(* Logix 5000 AddOnInstructionDefinition export MAJ_Yaskawa; software revision 17.00 *)

TYPE Yaskawa_EIP_Servo :   // Yaskawa SigmaLogic Axis Structure v2.4.0
STRUCT
   O : Yaskawa_OUT_to_Servo;
   I : Yaskawa_IN_from_Servo;
   AOI_SB : Yaskawa_AOI_Status_Bits;
END_STRUCT
END_TYPE

TYPE Yaskawa_OUT_to_Servo :   // Structure of data sent out to the Yaskawa SigmaLogic controller v2.4.0
STRUCT
   b00_ServoOn : BOOL;   // Servo On
   b01_Stop : BOOL;   // Stops All Current Motion in Progress
   b02_Home : BOOL;   // Start Homing Process
   b03_MoveStart1 : BOOL;   // Start Current Motion
   b06_SuperImpose : BOOL;
   b07_ServoAlarmReset : BOOL;   // Servo Alarm Reset
   b08_ControllerAlarmReset : BOOL;   // SigmaLogic Alarm Reset
   b09_MoveStart2 : BOOL;   // Start Second Motion (Blended Move)
   b10_MoveAbort : BOOL;   // Abort Current Move
   b11_MovePause : BOOL;   // Pause Current Move
   b12_SeqPause : BOOL;   // Indexing Sequence Pause
   b13_SeqResume : BOOL;   // Indexing Sequence Resume
   b14_SeqCancel : BOOL;   // Indexing Sequence Cancel
   b15_AbsEncoderReset : BOOL;   // Absolute Encoder Reset
   b16_SeqStart : BOOL;   // Start Indexing Sequence
   b17_SeqEditSpeed : BOOL;   // Enter Edit Speed
   b18_SeqEditDistance : BOOL;   // Enter Distance Edit
   b19_PLSEnable : BOOL;   // Enable PLS execution
   b20_PLSActivateOutput1 : BOOL;   // Activate PLS output1 switch logic
   b21_PLSActivateOutput2 : BOOL;   // Activate PLS output2 switch logic
   b22_PLSActivateOutput3 : BOOL;   // Activate PLS output3 switch logic
   b23_PLSActivateOutput4 : BOOL;   // Activate PLS output4 switch logic
   b24_SetClock : BOOL;   // Set the remote controller clock with data provided by the PLC
   RebootController : BOOL;
   UseExternalEncoder : BOOL;   // Use External Encoder when executing MAHSP_Yaskawa
   b32_HeatbeatAnswer : BOOL;   // Heartbeat Answer
   BrakeBypassRequest : BOOL;
   SetFwdTorqueLimit : BOOL;
   SetRevTorqueLimit : BOOL;
   TorqueLimit : DINT;
   TorqueRamp : DINT;
   HomeMethod : INT;
   HomeSpeed : DINT;
   HomeAccDec : DINT;   // Home Move Acceleration/Deceleration Rate
   HomeBackOffDistance : DINT;
   HomeCreepSpeed : DINT;
   HomeCreepDistanceLimit : DINT;
   HomeCreepTimeLimit : DINT;
   HomeOffsetDistance : DINT;
   HomeOffsetSpeed : DINT;
   HomePostion : DINT;
   HomeTorque : DINT;
   HomeInputNo : DINT;
   HomeApproachTimeLimit : DINT;
   HomeApproachDistLimit : DINT;
   HomeDirection : INT;
   HomeSwitchMode : INT;
   MoveType : INT;
   MoveDirection : INT;
   MoveAccel1 : DINT;
   MoveAccel2 : DINT;
   MoveDecel1 : DINT;
   MoveDecel2 : DINT;
   MoveSpeed1 : DINT;
   MoveSpeed2 : DINT;
   MoveDistance1 : DINT;
   MoveDistance2 : DINT;
   MovePosition1 : DINT;
   MovePosition2 : DINT;
   RegistrationDistance : DINT;
   GearNumerator : DINT;
   GearDenominator : DINT;
   SuperImposeDistance : DINT;
   Resolution : INT;
   RegistrationDirection : INT;
   TuningLevel : INT;
   SequenceStep : INT;   // Staring Sequence Step Number
   SequenceEditStep : INT;   // Sequence Step Number to Edit
   FlagCommandBits1 : DINT;   // Flag Commands. 1..64 are General Flags, Bits 0..31 correspond to Flag 1..32
   FlagCommandBits2 : DINT;   // Flag Commands cont. 1..64 are General Flags, Bits 0..31 correspond to Flag 33..64
   DigitalOutCommandBits : DINT;   // Digital Output commands. Bits 0-7 correspond to CN13 Digital Outputs 0-7, used as Flag 73-80. Bits 8-10 correspond to CN1 Digital Outputs 0-2 used as Flag 88-90"
   SequenceEditSpeed : DINT;
   SequenceEditDistance : DINT;
   FeedRateOverride : INT;
   HSI_Enable : BOOL;
   HSI_MoveMode : BOOL;   // 0=Relative; 1=Moves per Cycle
   HSI_CalcMethod : BOOL;   // 0=Accel/Decel; 1=Time
   HSI_MoveDirection : BOOL;   // 0 = Negative; 1 = Positive
   HSI_TriggerFlag : INT;
   HSI_MovingFlag : INT;
   HSI_DwellingFlag : INT;
   HSI_DoneFlag : INT;
   HSI_MoveType : INT;   // 0=Single; 1=Repeat; 2=Repeat "x" times
   HSI_RepeatNumber : INT;
   HSI_Distance : DINT;
   HSI_Speed : DINT;
   HSI_Accel : DINT;
   HSI_MoveTime : DINT;
   HSI_DwellTime : DINT;
   PLS_OutputFlag1 : INT;
   PLS_OutputFlag2 : INT;
   PLS_OutputFlag3 : INT;
   PLS_OutputFlag4 : INT;
   PLS_OnPosition1 : DINT;
   PLS_OffPosition1 : DINT;
   PLS_OnPosition2 : DINT;
   PLS_OffPosition2 : DINT;
   PLS_OnPosition3 : DINT;
   PLS_OffPosition3 : DINT;
   PLS_OnPosition4 : DINT;
   PLS_OffPosition4 : DINT;
   PLS_OnCompensation1 : INT;
   PLS_OffCompensation1 : INT;
   PLS_OnCompensation2 : INT;
   PLS_OffCompensation2 : INT;
   PLS_OnCompensation3 : INT;
   PLS_OffCompensation3 : INT;
   PLS_OnCompensation4 : INT;
   PLS_OffCompensation4 : INT;
   RTC_Year : INT;
   RTC_Month : INT;
   RTC_Day : INT;
   RTC_Hour : INT;
   RTC_Min : INT;
   RTC_Sec : INT;
   StopDecel : DINT;
   AnalogOutput : INT;   // CN13, AO_01 [mV]
END_STRUCT
END_TYPE

TYPE Yaskawa_AOI_Status_Bits :   // Internal bits used to interlock Yaskawa AOI execution. v2.4.0
STRUCT
   MAM : BOOL;   // Move AOI Active
   MAJ : BOOL;   // Jog AOI Active
   MAB : BOOL;   // Blending AOI Active
   MAG : BOOL;   // Gearing AOI Active
   MAHSP : BOOL;   // Home SetPoint AOI Active
   MAH : BOOL;   // Homing AOI Active
   MSQE : BOOL;   // Sequence Edit AOI Active
   MSQR : BOOL;   // Sequence Run AOI Active
   MHSI : BOOL;   // High Speed Index AOI Active
   MSO : BOOL;   // Servo On
   MSF : BOOL;   // Servo Off
   MAFR : BOOL;   // Fault Reset
   MAS : BOOL;   // Servo Abort
   MTRQ : BOOL;   // Torque Mode Active
   MPLS : BOOL;   // PLS Active
   MCLK : BOOL;   // SetClock Active
   MSTL : BOOL;   // Set Torque Limit Active
   AOI_Permissive : BOOL;   // Permissive to Execute an AOI
END_STRUCT
END_TYPE

TYPE Yaskawa_IN_from_Servo :   // Structure of data coming from the Yaskawa SigmaLogic controller. v2.4.0
STRUCT
   AlarmText : STRING;   // ServoPack Alarm Code plus Text Description
   b00_Heartbeat : BOOL;
   b01_Alarm : BOOL;   // ServoPack Alarm
   b02_Warning : BOOL;   // ServoPack Warning
   b03_Ready : BOOL;   // ServoPack Ready
   b04_Enabled : BOOL;   // ServoPack Enabled ("Servo On")
   b05_StopComplete : BOOL;
   b06_HomeComplete : BOOL;
   b07_HomeBusy : BOOL;
   b08_HomeActive : BOOL;
   b09_HomeAborted : BOOL;
   b10_HomeError : BOOL;
   b11_MoveAbsComplete : BOOL;
   b12_MoveAbsBusy : BOOL;
   b13_MoveAbsActive : BOOL;
   b14_MoveAbsAborted : BOOL;
   b15_MoveAbsError : BOOL;
   b16_MoveRelComplete : BOOL;
   b17_MoveRelBusy : BOOL;
   b18_MoveRelActive : BOOL;
   b19_MoveRelAborted : BOOL;
   b20_MoveRelError : BOOL;
   b21_JogAtSpeed : BOOL;
   b22_JogBusy : BOOL;
   b23_JogActive : BOOL;
   b24_JogAborted : BOOL;
   b25_JogError : BOOL;
   b26_GearInSync : BOOL;
   b27_GearBusy : BOOL;
   b28_GearActive : BOOL;
   b29_GearAborted : BOOL;
   b30_GearError : BOOL;
   b32_MoveSuperComplete : BOOL;
   b33_MoveSuperBusy : BOOL;
   b34_MoveSuperActive : BOOL;
   b35_MoveSuperAborted : BOOL;
   b36_MoveSuperError : BOOL;
   b37_PowerCycleRequired : BOOL;
   b38_MoveBlend1Complete : BOOL;
   b39_MoveBlend1Busy : BOOL;
   b40_MoveBlend1Active : BOOL;
   b41_MoveBlend1Abort : BOOL;
   b42_MoveBlend1Error : BOOL;
   b43_MoveBlend2Complete : BOOL;
   b44_MoveBlend2Busy : BOOL;
   b45_MoveBlend2Active : BOOL;
   b46_MoveBlend2Abort : BOOL;
   b47_MoveBlend2Error : BOOL;
   b48_RegComplete : BOOL;
   b49_RegBusy : BOOL;
   b50_RegActive : BOOL;
   b51_RegAborted : BOOL;
   b52_RegError : BOOL;
   b53_ResetAbsEncoderActive : BOOL;
   b54_ResetAbsEncoderBusy : BOOL;
   b55_ResetAbsEncoderDone : BOOL;
   b56_ResetAbsEncoderError : BOOL;
   b57_SeqRunning : BOOL;
   b58_RegSensorNotReached : BOOL;
   b59_SeqEditError : BOOL;
   b60_SeqEditDone : BOOL;
   b61_TorqueAtTorque : BOOL;
   b62_TorqueBusy : BOOL;
   b63_TorqueActive : BOOL;
   b64_TorqueAborted : BOOL;
   b65_TorqueError : BOOL;
   b66_ControllerAlarm : BOOL;
   b67_ApplicationError : BOOL;
   b68_AxisAtStandStill : BOOL;
   b69_TestModeActive : BOOL;
   b70_ServoParamsOK : BOOL;
   b71_SetFwdTorqueLimitDone : BOOL;
   b72_SetRevTorqueLimitDone : BOOL;
   Position : DINT;
   Speed : DINT;
   Torque : DINT;
   HomeErrorID : INT;
   MoveAbsErrorID : INT;
   MoveRelErrorID : INT;
   JogErrorID : INT;
   GearErrorID : INT;
   MoveSuperErrorID : INT;
   ServoAlarmID : INT;
   ServoWarningID : INT;
   ControllerAlarmID : DINT;
   AxisGenAlarmID : DINT;
   MoveBlend1ErrorID : INT;
   MoveBlend2ErrorID : INT;
   ResetAbsEncoderErrorID : INT;
   FunctionBlockErrorID : INT;
   TorqueErrorID : INT;
   RegErrorID : INT;
   SeqCurrentStep : INT;
   FlagStatusBit1 : DINT;   // Flag Status. 1..64 are General Flags, Bits 0..31 correspond to Flag 1..32
   FlagStatusBit2 : DINT;   // Flag Status cont. 1..64 are General Flags, Bits 0..31 correspond to Flag 33..64
   IOStatusBits : DINT;   // Digital IO Status. Bits 0-7, CN13 Inputs 0-7, Used as Flag 65-72. Bits 8-15, CN13 Outputs 0-7, Used as Flag 73-80. Bits 16-22, CN1 Inputs 0-6, Used as Flag 81-87. Bits 23-25, CN1 Outputs 0-4, Used as Flag 88-92.
   HSI_Moving : BOOL;
   HSI_Dwelling : BOOL;
   HSI_Done : BOOL;
   HSI_Busy : BOOL;
   HSI_Error : BOOL;
   HSI_ErrorCode : INT;
   PLS_Running : BOOL;
   PLS_SwitchStatus1 : BOOL;
   PLS_SwitchStatus2 : BOOL;
   PLS_SwitchStatus3 : BOOL;
   PLS_SwitchStatus4 : BOOL;
   PLS_Busy : BOOL;
   PLS_Error : BOOL;
   PLS_ErrorCode : INT;
   SetClock_Done : BOOL;
   SetClock_Busy : BOOL;
   SetClock_Error : BOOL;
   SetClock_ErrorID : INT;
   SoftwareVersion : DINT;
   FirmwareVersion : DINT;
   CommandedPos : DINT;
   CommandedPosNonCyc : DINT;
   CommandedSpeed : DINT;
   Clock_Year : INT;
   Clock_Month : INT;
   Clock_Day : INT;
   Clock_Hour : INT;
   Clock_Minute : INT;
   Clock_Second : INT;
   AnalogInput : REAL;   // CN13, AI_01 [v]
   BrakeBypassActive : BOOL;
   ForwardTorqueLimit : DINT;
   ReverseTorqueLimit : DINT;
END_STRUCT
END_TYPE

ADD_ON_INSTRUCTION MAJ_Yaskawa   (* revision 2.4 0, vendor Yaskawa America, Inc., ExecuteEnableInFalse *)
// Motion Axis Jog
// Revision note:
// 2.4.0: No functional change
// 2.3.1: Moved unlatch of AOI_ON_LOCAL to bottom of EnableInFalse routine so that outputs will be on for at least 1 scan upon completion.
// 2.3.0: No functional change
// 2.0.0: Improved output operation and error code reporting. Improved interlocking with embedded code.
// 1.2.0: No functional change.
// Initial Release 9/10/2014
// Help:
// This AOI moves a servo axis indefinitely at a commanded speed based on the motion profile parameters. Use the Motion Axis Jog instruction to jog the axis with or without registration. Speed may be updated on-the-fly without stopping by changing the value for Speed while holding the block EnableIN input ON.
// When the MAJ_Yaskawa EnableIN is removed, the axis will decelerate to a stop - no need to activate the MAS_Yaskawa command separately.
VAR_IN_OUT
   Axis : Yaskawa_EIP_Servo; {required}
END_VAR
VAR_INPUT
   Direction : INT; {required}   // 0 = Forward 1 = Reverse
   Speed : REAL; {required}   // Commanded Speed [unit/s]
   Accel_Rate : REAL; {required}   // Acceleration rate [unit/s/s]
   Decel_Rate : REAL; {required}   // Deceleration rate [unit/s/s]
   RegistrationUse : INT; {required}   // 0 = Disabled (Do Not use Registration Latch) 1 = Enabled (Arm the Registration Latch)
   Reg_Distance : REAL; {required}   // Registration Distance to Move (Relative)
   Reg_Speed : REAL; {required}   // Registration Move Speed [unit/s]
   Reg_Accel : REAL; {required}   // Registration Move Acceleration rate [unit/s/s]
   Reg_Decel : REAL; {required}   // Registration Move Deceleration rate [unit/s/s]
END_VAR
VAR_OUTPUT
   EN : BOOL; {visible}   // The AOI is Active
   DN : BOOL; {visible}   // Jog motion has been initiated
   IP : BOOL; {visible}   // Axis jog motion is In Process
   ER : BOOL; {visible}   // Jog Motion Error
   PC : BOOL; {visible}   // The axis is jogging at commanded speed
   RegDN : BOOL; {visible}   // Registration move has been initiated
   RegIP : BOOL; {visible}   // The Axis is moving to the Registration Position
   RegPC : BOOL; {visible}   // The Axis has reached the Registration Position
   FLT_RDY : BOOL; {visible}   // The Servo is Not Ready
   FLT_BSY : BOOL; {visible}   // There is another AOI Active for this Axis
   ErrorCode : INT; {visible}   // Jog Error Code
   RegErrorCode : INT; {visible}   // Registration Move Error Code
END_VAR
VAR
   AOI_ON_LOCAL : BOOL;
   Move_JOG : BOOL;
   Move_JOG_wREG : BOOL;
   ScaleFactor : DINT;
   Execute_OS : BOOL;
   Finished : BOOL;   // Function is finished
   Stopping : BOOL;
END_VAR

ROUTINE EnableInFalse   (* ladder *)
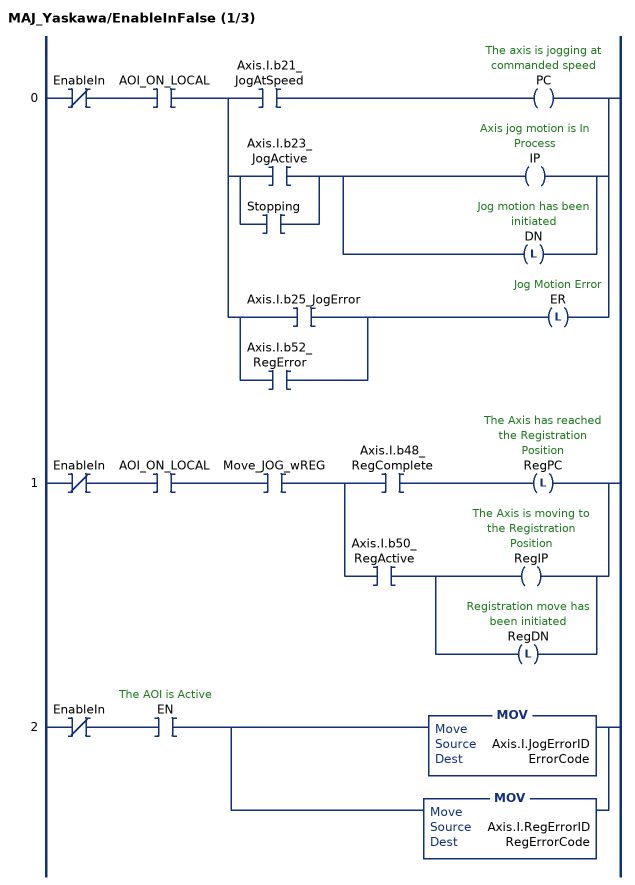
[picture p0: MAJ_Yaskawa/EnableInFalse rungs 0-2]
   0: XIO(EnableIn)XIC(AOI_ON_LOCAL)[XIC(Axis.I.b21_JogAtSpeed) OTE(PC) ,[XIC(Axis.I.b23_JogActive) ,XIC(Stopping) ] [OTE(IP) ,OTL(DN) ] ,[XIC(Axis.I.b25_JogError) ,XIC(Axis.I.b52_RegError) ] OTL(ER) ];
   1: XIO(EnableIn)XIC(AOI_ON_LOCAL)XIC(Move_JOG_wREG)[XIC(Axis.I.b48_RegComplete) OTL(RegPC) ,XIC(Axis.I.b50_RegActive) [OTE(RegIP) ,OTL(RegDN) ] ];
   2: XIO(EnableIn)XIC(EN)[MOV(Axis.I.JogErrorID,ErrorCode) ,MOV(Axis.I.RegErrorID,RegErrorCode) ];
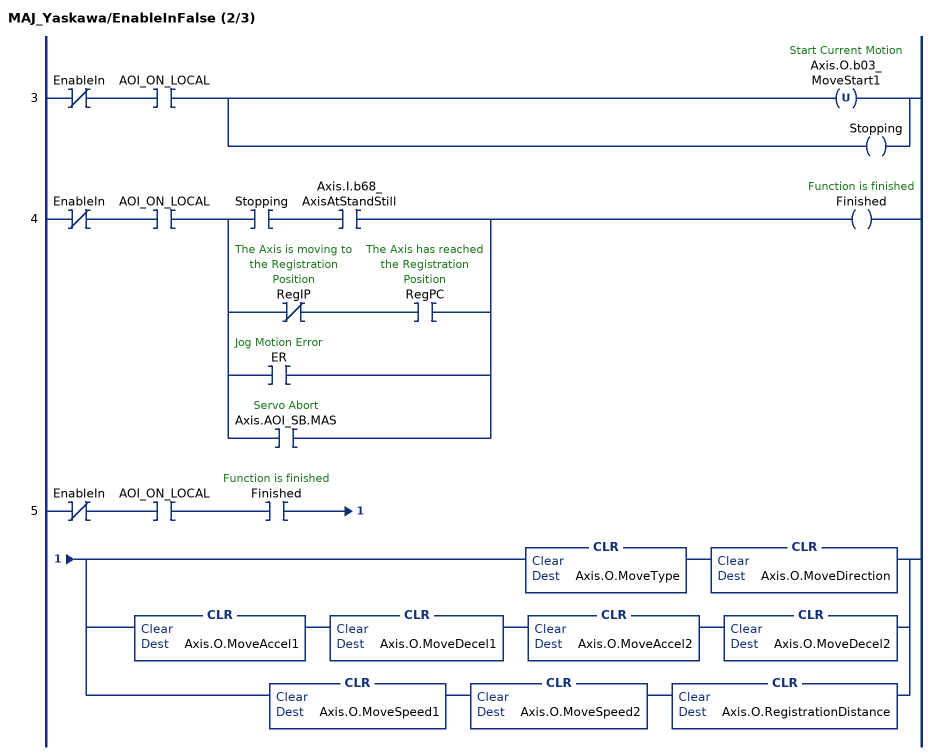
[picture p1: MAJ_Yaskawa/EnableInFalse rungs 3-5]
   3: XIO(EnableIn)XIC(AOI_ON_LOCAL)[OTU(Axis.O.b03_MoveStart1) ,OTE(Stopping) ];
   4: XIO(EnableIn)XIC(AOI_ON_LOCAL)[XIC(Stopping) XIC(Axis.I.b68_AxisAtStandStill) ,XIO(RegIP) XIC(RegPC) ,XIC(ER) ,XIC(Axis.AOI_SB.MAS) ]OTE(Finished);
   5: XIO(EnableIn)XIC(AOI_ON_LOCAL)XIC(Finished)[CLR(Axis.O.MoveType) CLR(Axis.O.MoveDirection) ,CLR(Axis.O.MoveAccel1) CLR(Axis.O.MoveDecel1) CLR(Axis.O.MoveAccel2) CLR(Axis.O.MoveDecel2) ,CLR(Axis.O.MoveSpeed1) CLR(Axis.O.MoveSpeed2) CLR(Axis.O.RegistrationDistance) ];
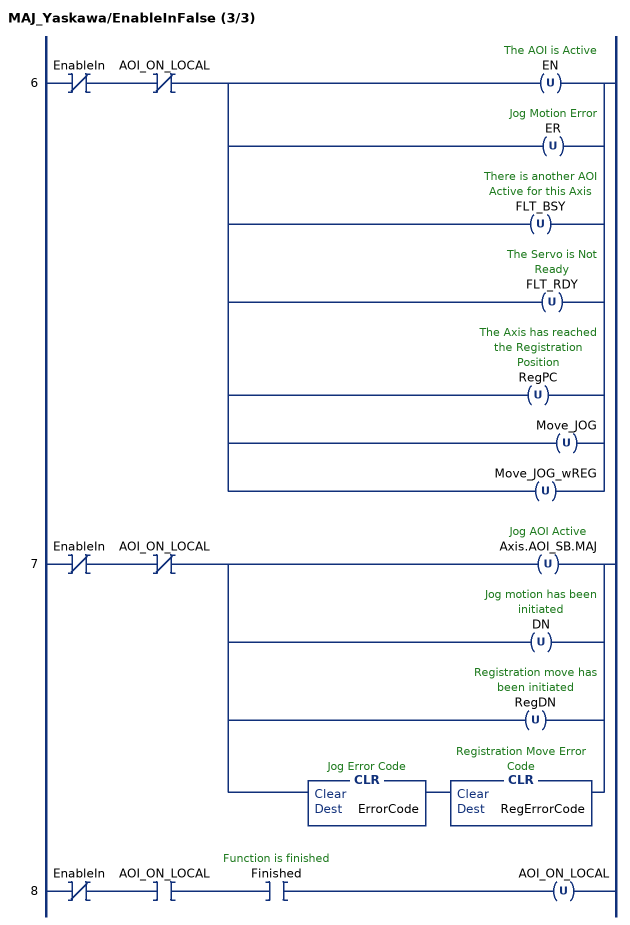
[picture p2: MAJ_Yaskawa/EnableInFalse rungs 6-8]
   6: XIO(EnableIn)XIO(AOI_ON_LOCAL)[OTU(EN) ,OTU(ER) ,OTU(FLT_BSY) ,OTU(FLT_RDY) ,OTU(RegPC) ,OTU(Move_JOG) ,OTU(Move_JOG_wREG) ];
   7: XIO(EnableIn)XIO(AOI_ON_LOCAL)[OTU(Axis.AOI_SB.MAJ) ,OTU(DN) ,OTU(RegDN) ,CLR(ErrorCode) CLR(RegErrorCode) ];
   8: XIO(EnableIn)XIC(AOI_ON_LOCAL)XIC(Finished)OTU(AOI_ON_LOCAL);
END_ROUTINE

ROUTINE Logic   (* ladder *)
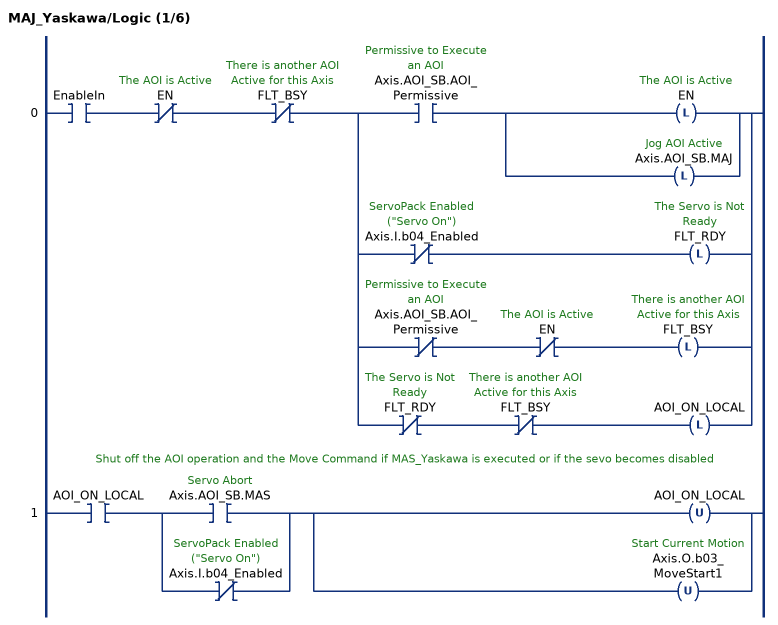
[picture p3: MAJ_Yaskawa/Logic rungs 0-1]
   0: XIC(EnableIn)XIO(EN)XIO(FLT_BSY)[XIC(Axis.AOI_SB.AOI_Permissive) [OTL(EN) ,OTL(Axis.AOI_SB.MAJ) ] ,XIO(Axis.I.b04_Enabled) OTL(FLT_RDY) ,XIO(Axis.AOI_SB.AOI_Permissive) XIO(EN) OTL(FLT_BSY) ,XIO(FLT_RDY) XIO(FLT_BSY) OTL(AOI_ON_LOCAL) ];
   // Shut off the AOI operation and the Move Command if MAS_Yaskawa is executed or if the sevo becomes disabled
   1: XIC(AOI_ON_LOCAL)[XIC(Axis.AOI_SB.MAS) ,XIO(Axis.I.b04_Enabled) ][OTU(AOI_ON_LOCAL) ,OTU(Axis.O.b03_MoveStart1) ];
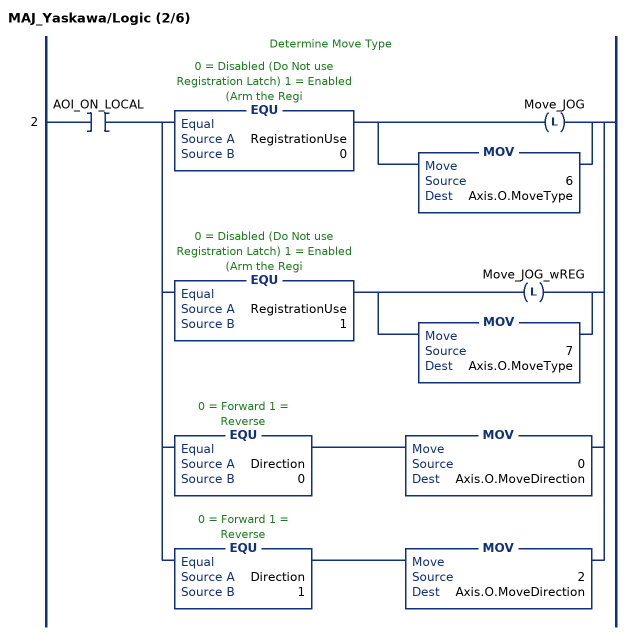
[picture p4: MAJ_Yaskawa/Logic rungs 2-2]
   // Determine Move Type
   2: XIC(AOI_ON_LOCAL)[EQU(RegistrationUse,0) [OTL(Move_JOG) ,MOV(6,Axis.O.MoveType) ] ,EQU(RegistrationUse,1) [OTL(Move_JOG_wREG) ,MOV(7,Axis.O.MoveType) ] ,EQU(Direction,0) MOV(0,Axis.O.MoveDirection) ,EQU(Direction,1) MOV(2,Axis.O.MoveDirection) ];
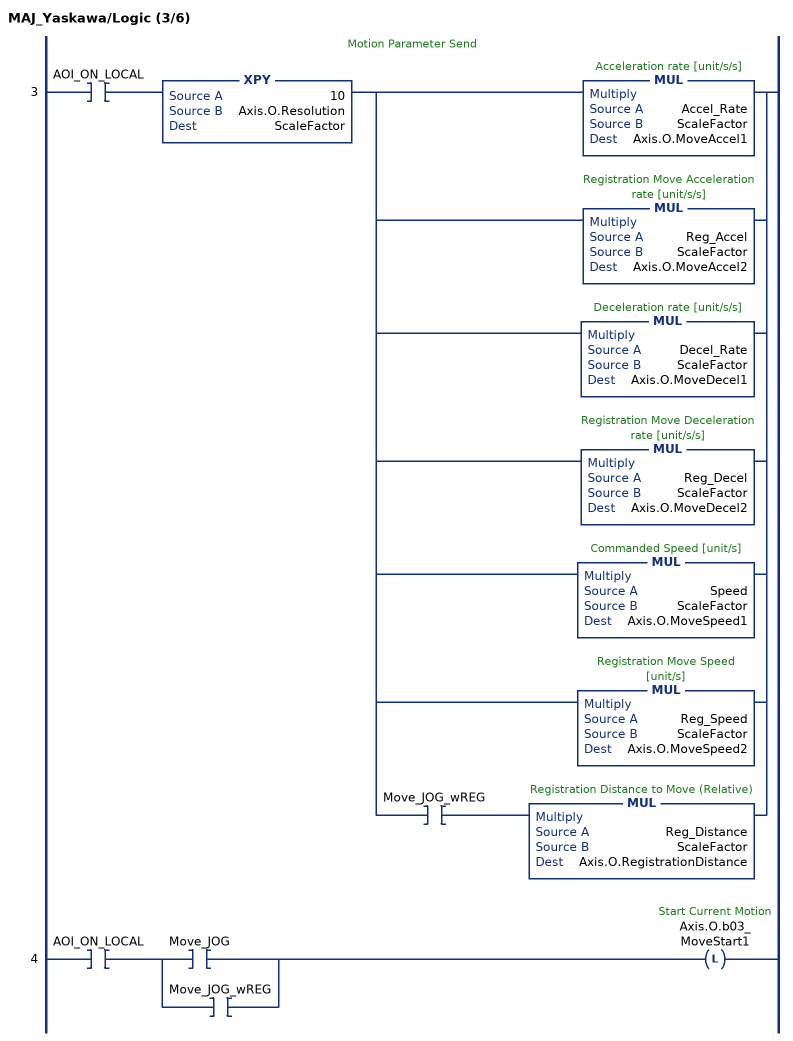
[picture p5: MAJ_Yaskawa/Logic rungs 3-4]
   // Motion Parameter Send
   3: XIC(AOI_ON_LOCAL)XPY(10,Axis.O.Resolution,ScaleFactor)[MUL(Accel_Rate,ScaleFactor,Axis.O.MoveAccel1) ,MUL(Reg_Accel,ScaleFactor,Axis.O.MoveAccel2) ,MUL(Decel_Rate,ScaleFactor,Axis.O.MoveDecel1) ,MUL(Reg_Decel,ScaleFactor,Axis.O.MoveDecel2) ,MUL(Speed,ScaleFactor,Axis.O.MoveSpeed1) ,MUL(Reg_Speed,ScaleFactor,Axis.O.MoveSpeed2) ,XIC(Move_JOG_wREG) MUL(Reg_Distance,ScaleFactor,Axis.O.RegistrationDistance) ];
   4: XIC(AOI_ON_LOCAL)[XIC(Move_JOG) ,XIC(Move_JOG_wREG) ]OTL(Axis.O.b03_MoveStart1);
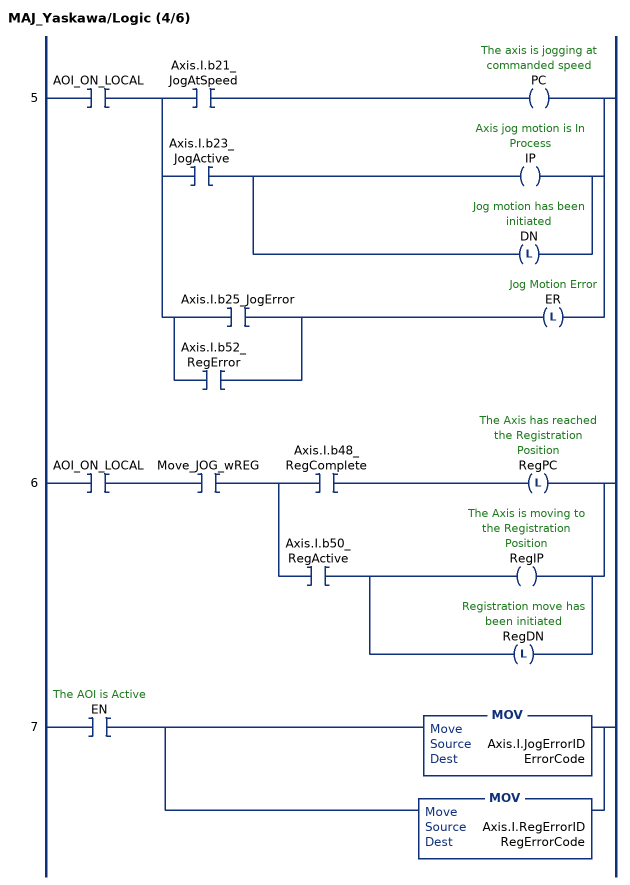
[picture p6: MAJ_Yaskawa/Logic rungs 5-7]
   5: XIC(AOI_ON_LOCAL)[XIC(Axis.I.b21_JogAtSpeed) OTE(PC) ,XIC(Axis.I.b23_JogActive) [OTE(IP) ,OTL(DN) ] ,[XIC(Axis.I.b25_JogError) ,XIC(Axis.I.b52_RegError) ] OTL(ER) ];
   6: XIC(AOI_ON_LOCAL)XIC(Move_JOG_wREG)[XIC(Axis.I.b48_RegComplete) OTL(RegPC) ,XIC(Axis.I.b50_RegActive) [OTE(RegIP) ,OTL(RegDN) ] ];
   7: XIC(EN)[MOV(Axis.I.JogErrorID,ErrorCode) ,MOV(Axis.I.RegErrorID,RegErrorCode) ];
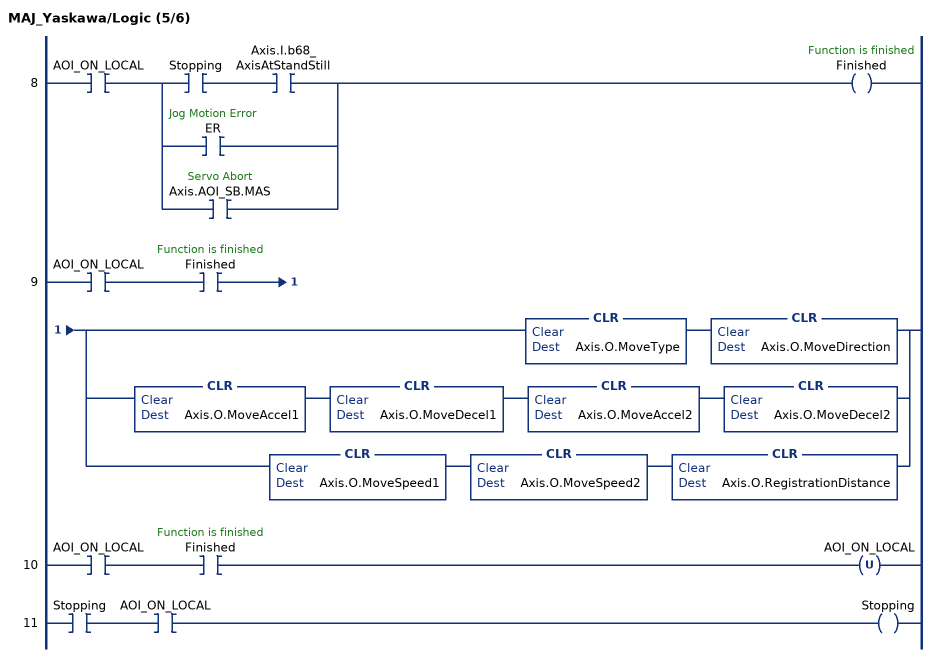
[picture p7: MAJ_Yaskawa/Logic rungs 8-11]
   8: XIC(AOI_ON_LOCAL)[XIC(Stopping) XIC(Axis.I.b68_AxisAtStandStill) ,XIC(ER) ,XIC(Axis.AOI_SB.MAS) ]OTE(Finished);
   9: XIC(AOI_ON_LOCAL)XIC(Finished)[CLR(Axis.O.MoveType) CLR(Axis.O.MoveDirection) ,CLR(Axis.O.MoveAccel1) CLR(Axis.O.MoveDecel1) CLR(Axis.O.MoveAccel2) CLR(Axis.O.MoveDecel2) ,CLR(Axis.O.MoveSpeed1) CLR(Axis.O.MoveSpeed2) CLR(Axis.O.RegistrationDistance) ];
   10: XIC(AOI_ON_LOCAL)XIC(Finished)OTU(AOI_ON_LOCAL);
   11: XIC(Stopping)XIC(AOI_ON_LOCAL)OTE(Stopping);
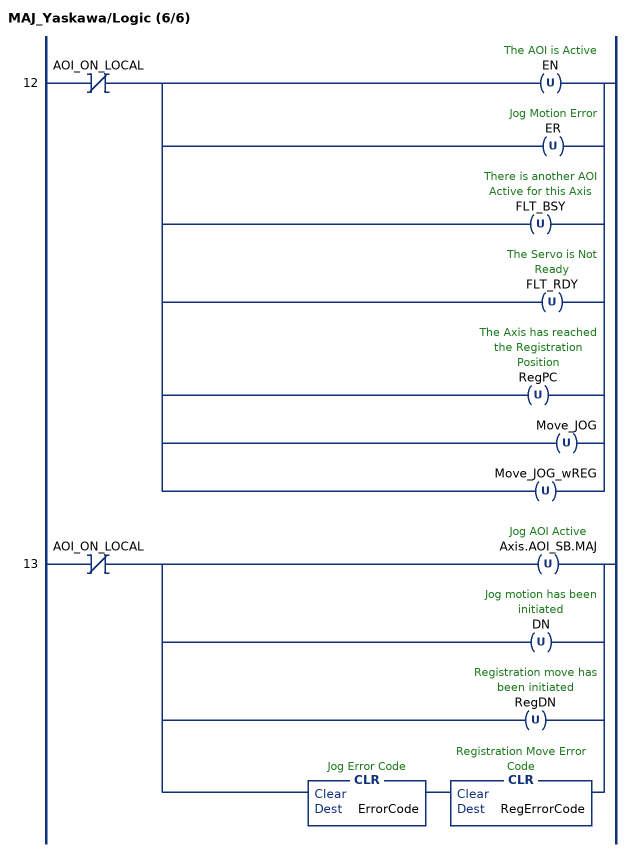
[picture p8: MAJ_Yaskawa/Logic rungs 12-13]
   12: XIO(AOI_ON_LOCAL)[OTU(EN) ,OTU(ER) ,OTU(FLT_BSY) ,OTU(FLT_RDY) ,OTU(RegPC) ,OTU(Move_JOG) ,OTU(Move_JOG_wREG) ];
   13: XIO(AOI_ON_LOCAL)[OTU(Axis.AOI_SB.MAJ) ,OTU(DN) ,OTU(RegDN) ,CLR(ErrorCode) CLR(RegErrorCode) ];
END_ROUTINE
END_ADD_ON_INSTRUCTION
